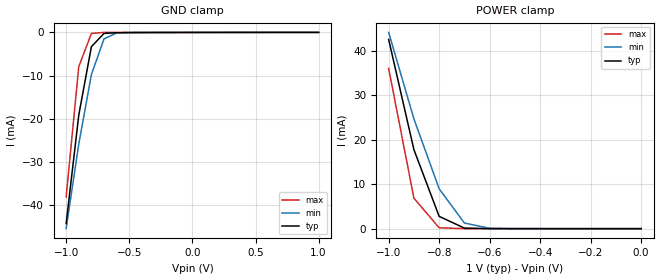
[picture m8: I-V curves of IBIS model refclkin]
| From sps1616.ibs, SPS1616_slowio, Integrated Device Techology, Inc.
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|   Model refclkin
[Model]   refclkin
Model_type   Terminator
Polarity   Non-Inverting
C_comp   0.2000pF   0.2000pF   0.2000pF
[Temperature Range]   62.5000   0.1250k   0.000
[Voltage Range]   1.0000V   0.9000V   1.1000V
[Rpower]   83.9   80.8   87.6
[Rgnd]   175   256   136
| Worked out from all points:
|   GND clamp passes 1 mA (typ) near -0.72 V on its own axis
|   POWER clamp passes 1 mA (typ) near -0.73 V on its own axis
[GND_clamp]
| voltage   I(typ)   I(min)   I(max)
-1V       -44.28mA   -45.46mA   -38.12mA
-900mV    -19.15mA   -25.85mA   -7.919mA
-800mV    -3.311mA   -9.764mA   -245.1uA
-700mV    -237.1uA   -1.501mA   -4.402uA
-600mV    -76.55uA   -124uA     -427.2nA
-500mV    -57.06uA   -25.18uA   -286.8nA
1V        0A         0A         0A
[POWER_clamp]
| voltage   I(typ)   I(min)   I(max)
-1V       42.61mA    44.19mA    36.07mA
-900mV    17.8mA     24.73mA    6.876mA
-800mV    2.772mA    8.973mA    195.4uA
-700mV    124.1uA    1.272mA    4.006uA
-600mV    4.543uA    84.02uA    643.7nA
-500mV    343nA      4.937uA    383.2nA
-400mV    128nA      341.2nA    238.7nA
-300mV    0A         0A         143.9nA
-200mV    0A         0A         0A
0V        0A         0A         0A
